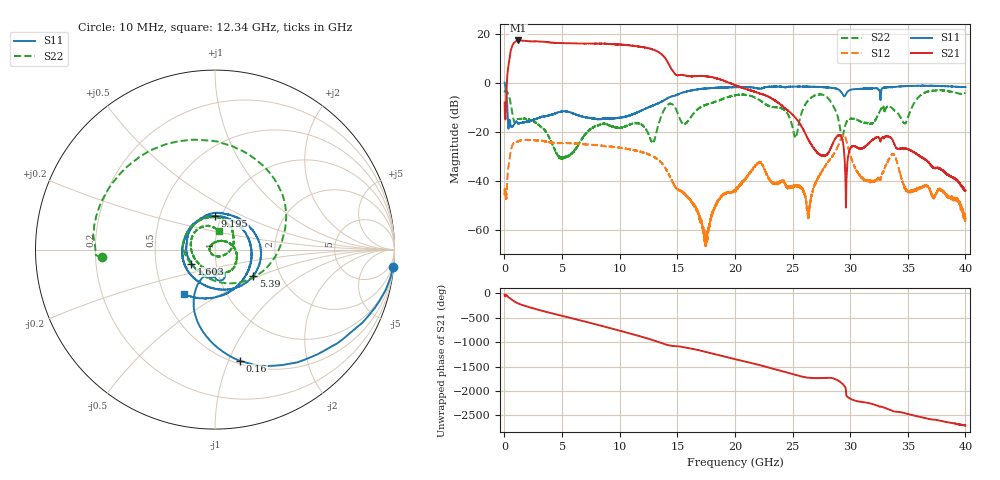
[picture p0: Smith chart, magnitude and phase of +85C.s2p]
!Agilent Technologies,E8363C,MY49030334,A.09.42.15
!Agilent E8363C: A.09.42.15
!Date: Thursday, February 26, 2026 09:47:58
!Correction: S11(Full 2 Port(1,2))
!S21(Full 2 Port(1,2))
!S12(Full 2 Port(1,2))
!S22(Full 2 Port(1,2))
!S2P File: Measurements: S11, S21, S12, S22:
# Hz S  dB  R 50
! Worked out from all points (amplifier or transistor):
!   6401 points, 10 MHz to 40 GHz, reference 50 ohm
!   highest |S21| = 17.2 dB at 1.203 GHz (marker M1)
!   |S21| within 3 dB of that: 615.4 MHz to 12.33 GHz (11.71 GHz wide, 181 % of centre)
!   unconditionally stable (mu >= 1): 13.08 MHz to end of sweep
!   at 6.671 GHz: K = 1.54, MAG = 16.2 dB, |S12| = -25.1 dB
!   at 20 GHz: K = 21.83, MAG = 5.1 dB, |S12| = -44.1 dB
!   at 40 GHz: K = 9873.90, MAG = -37.0 dB, |S12| = -55.7 dB
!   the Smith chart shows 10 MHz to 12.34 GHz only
!   S11 on the Smith chart (normalised r, x): 10 MHz: 0, -21; 160 MHz: 0.53, -1.10; 1.603 GHz: 0.76, -0.12; 5.39 GHz: 1.45, -0.46; 9.195 GHz: 0.93, +0.36; 12.34 GHz: 0.63, -0.34
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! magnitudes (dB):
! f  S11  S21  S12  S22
! 10 MHz  0.0  -8.2  -43.4  -4.0
! 160 MHz  -3.9  -5.3  -47.4  -3.5
! 572.4 MHz  -18.1  13.5  -27.2  -9.4
! 1.203 GHz  -16.7  17.2  -23.9  -14.8
! 1.603 GHz  -16.3  17.1  -23.4  -14.7
! 5.39 GHz  -11.8  16.1  -24.6  -30.1
! 6.677 GHz  -13.8  15.9  -25.1  -23.2
! 9.195 GHz  -14.5  15.7  -26.1  -17.6
! 12.34 GHz  -10.4  14.2  -28.9  -19.5
! 13.34 GHz  -8.4  12.5  -31.5  -17.5
! 17.43 GHz  -2.4  2.6  -64.3  -9.1
! 20 GHz  -1.9  -1.0  -44.1  -5.2
! 22.12 GHz  -2.4  -4.4  -32.5  -7.1
! 25.25 GHz  -1.6  -14.3  -42.0  -22.4
! 26.67 GHz  -1.7  -25.6  -45.7  -5.9
! 29.38 GHz  -5.1  -24.5  -21.4  -21.8
! 29.68 GHz  -4.3  -39.0  -23.9  -16.1
! 31.23 GHz  -2.5  -26.4  -39.7  -16.4
! 33.34 GHz  -1.9  -22.0  -31.4  -9.7
! 34.75 GHz  -1.4  -26.8  -42.9  -16.6
! 36.45 GHz  -1.3  -31.2  -41.9  -4.2
! 40 GHz  -1.8  -43.8  -55.7  -4.1
